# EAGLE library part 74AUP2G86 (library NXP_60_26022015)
Low-power dual 2-input EXCLUSIVE-OR gate The 74AUP2G86 provides the dual 2-input EXCLUSIVE-OR function. Schmitt trigger action at all inputs makes the circuit tolerant to slower input rise and fall times across the entire VCC range from 0.8 V to 3.6 V. This device ensures a very low static and dynamic power consumption across the entire VCC range from 0.8 V to 3.6 V. This device is fully specified for partial power-down applications using IOFF. The IOFF circuitry disables the output, preventing a damaging backflow current through the device when it is powered down. AAL Eindhoven MK
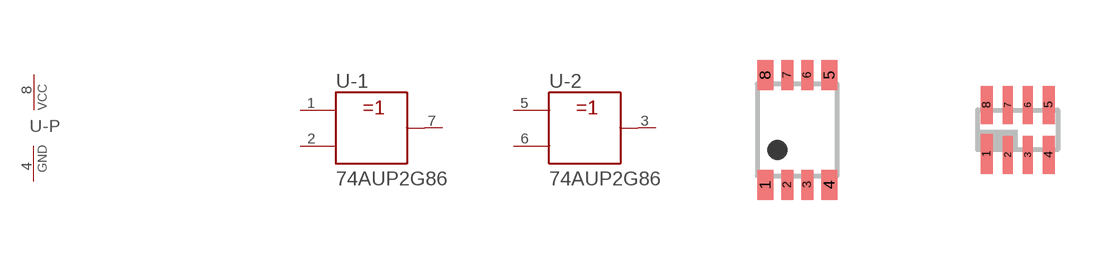
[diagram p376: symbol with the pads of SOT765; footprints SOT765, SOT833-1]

Designator prefix U; gates -1=2-INPUT-EXCLUSIVE-OR -2=2-INPUT-EXCLUSIVE-OR -P=PWRN

## 74AUP2G86DC  [SOT765]
1  -1:A  in
2  -1:B  in
3  -2:Y  out
4  -P:GND  pwr
5  -2:A  in
6  -2:B  in
7  -1:Y  out
8  -P:VCC  pwr

## 74AUP2G86GT  [SOT833-1]
Pads as for SOT765

## 74AUP2G86GF  [SOT1089-1]
Pads as for SOT765

## 74AUP2G86GD  [SOT996-2/3]
Pads as for SOT765

## 74AUP2G86GM  [SOT902-1/2/3]
1  -1:Y  out
2  -2:B  in
3  -2:A  in
4  -P:GND  pwr
5  -2:Y  out
6  -1:B  in
7  -1:A  in
8  -P:VCC  pwr

## 74AUP2G86GS  [SOT1203]
Pads as for SOT765

## Footprint SOT765 (pad centres in mm)
SOT765 VSSOP8: plastic very thin shrink small outline package; 8 leads; body width 2.3 mm JEDEC: MO-187 IEC: -- JEITA: --
smd 0.4 x 0.75: 1 -0.8,-1.375; 4 0.8,-1.375; 5 0.8,1.375; 8 -0.8,1.375
smd 0.3 x 0.75: 2 -0.25,-1.375; 3 0.25,-1.375; 6 0.25,1.375; 7 -0.25,1.375

## Footprint SOT833-1 (pad centres in mm)
SOT833-1 XSON8: plastic extremely thin small outline package; no leads; 8 terminals; body 1 x 1.95 x 0.5 mm JEDEC: MO-252 IEC: -- JEITA: --
smd 0.3 x 1: 1 -0.775,-0.6
smd 0.25 x 0.95: 2 -0.25,-0.625; 3 0.25,-0.625; 6 0.25,0.625; 7 -0.25,0.625
smd 0.3 x 0.95: 4 0.775,-0.625; 5 0.775,0.625; 8 -0.775,0.625

## Footprint SOT1089-1 (pad centres in mm)
SOT1089-1 XSON8: plastic, extremely thin small outline package; no leads; 8 terminals; body 1 x 1.35 x 0.5 mm JEDEC: -- IEC: -- JEITA: --
smd 0.15 x 0.5: 1 -0.525,-0.35; 2 -0.175,-0.35; 3 0.175,-0.35; 4 0.525,-0.35; 5 0.525,0.35; 6 0.175,0.35; 7 -0.175,0.35; 8 -0.525,0.35

## Footprint SOT996-2/3 (pad centres in mm)
SOT996-2/3 XSON8U: plastic extremely thin small outline package; no leads;8 terminals; UTLP based; body 3 x 2 x 0.5 mm JEDEC: IEC: -- JEITA: --
smd 0.25 x 1.1: 1 -0.75,-1.45
smd 0.25 x 1: 2 -0.25,-1.5; 3 0.25,-1.5; 4 0.75,-1.5; 5 0.75,1.5; 6 0.25,1.5; 7 -0.25,1.5; 8 -0.75,1.5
